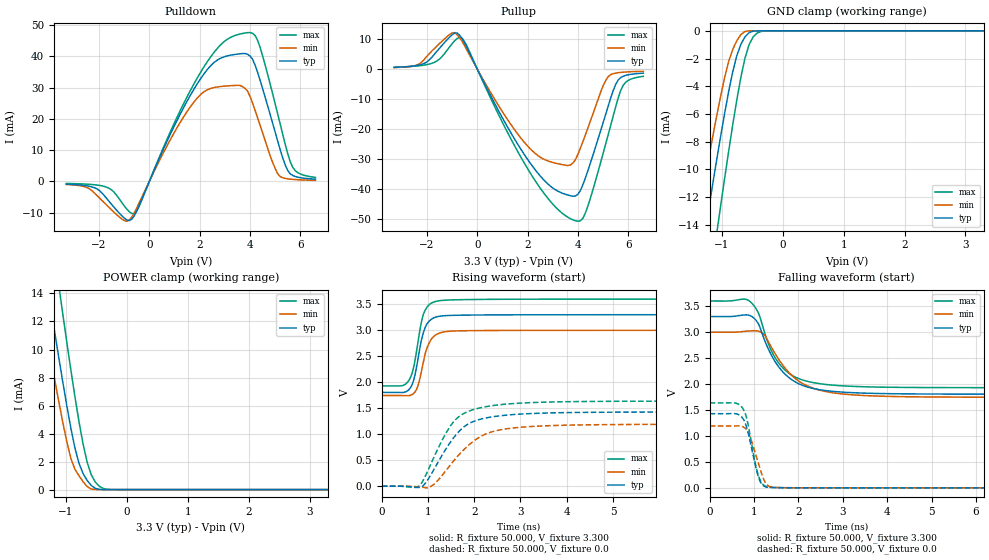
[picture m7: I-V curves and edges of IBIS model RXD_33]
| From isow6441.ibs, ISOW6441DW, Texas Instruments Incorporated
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|   RXD_33 Model
[Model]   RXD_33
Model_type 3-state
| Signals   RXD
Vmeas = 2.2V   |Reference voltage for timing measurements
Cref = 15pF   |Timing specification test load capacitance value
Vref = 0   |Timing specification test load voltage; GND
Polarity   Non-Inverting
Enable   Active-High
C_comp   2.100pF   1.700pF   2.500pF
[Temperature Range]   27.000   -40.000   0.125k
[Voltage Range]   3.300V   3.000V   3.600V
[Pullup Reference]   3.300V   3.000V   3.600V
[Pulldown Reference]   0.0V   0.0V   0.0V
[POWER Clamp Reference]   3.300V   3.000V   3.600V
[GND Clamp Reference]   0.0V   0.0V   0.0V
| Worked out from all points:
|   slope of the pulldown table from 0 to 0.495 V, typ, clamps not added: 54 ohm
|   slope of the pullup table from 0 to 0.495 V, typ, clamps not added: 59.6 ohm
|   GND clamp passes 1 mA (typ) near -0.69 V on its own axis
|   POWER clamp passes 1 mA (typ) near -0.70 V on its own axis
|   rising waveform, R_fixture 50.000, V_fixture 3.300: 20-80 % time 209ps typ, 218ps min, 204ps max; typ from 1.8 V to 3.3 V
|   rising waveform, R_fixture 50.000, V_fixture 0.0: 20-80 % time 673ps typ, 800ps min, 618ps max; typ from 0 V to 1.43 V
|   falling waveform, R_fixture 50.000, V_fixture 3.300: 20-80 % time 647ps typ, 760ps min, 564ps max; typ from 3.3 V to 1.8 V
|   falling waveform, R_fixture 50.000, V_fixture 0.0: 20-80 % time 231ps typ, 262ps min, 225ps max; typ from 1.43 V to 0 V
[Pulldown]
|Voltage   I(typ)   I(min)   I(max)
-3.3V     -873.2uA   -976.9uA   -658.3uA
-1.7V     -5.395mA   -7.539mA   -1.844mA
-900mV    -12.28mA   -12.75mA   -8.801mA
-600mV    -11.02mA   -10.11mA   -10.3mA
2V        32.38mA    27.46mA    34.36mA
3V        39.89mA    30.45mA    44.84mA
4V        40.06mA    27.17mA    47.56mA
4.4V      32.32mA    17.94mA    42.82mA
5.1V      12.87mA    2.427mA    21.53mA
5.5V      3.442mA    821uA      8.827mA
5.8V      1.561mA    581.2uA    3.422mA
6.6V      711uA      333.9uA    1.284mA
[Pullup]
|Voltage   I(typ)   I(min)   I(max)
-3.3V     572.5uA    495.9uA    587.7uA
-2.1V     1.91mA     3.303mA    1.333mA
-1V       11.42mA    12.06mA    8.45mA
-600mV    10.16mA    9.258mA    10.25mA
2.2V      -32.5mA    -27.4mA    -35.95mA
3.6V      -42.06mA   -32.22mA   -49.46mA
4V        -41.78mA   -28.45mA   -50.82mA
4.4V      -33.81mA   -19.56mA   -45.61mA
5.1V      -15.18mA   -3.859mA   -25.08mA
5.5V      -5.127mA   -1.348mA   -12.6mA
5.9V      -2.103mA   -980.9uA   -4.383mA
6.6V      -1.37mA    -744.9uA   -2.434mA
[GND_clamp]
|Voltage   I(typ)   I(min)   I(max)
-3.3V     -72.49mA   -60.83mA   -87.48mA
-1.424V   -18.62mA   -14.18mA   -25.42mA
-1.29V    -14.9mA    -10.95mA   -21.12mA
-1.223V   -13.05mA   -9.358mA   -18.98mA
-1.089V   -9.436mA   -6.249mA   -14.77mA
-1.022V   -7.681mA   -4.767mA   -12.71mA
-821mV    -2.955mA   -1.346mA   -6.782mA
-754mV    -1.794mA   -716.5uA   -4.976mA
-620mV    -433uA     -46.82uA   -1.974mA
-486mV    -22.19uA   -122.9nA   -439.7uA
-352mV    -188.7nA   -149.6pA   -41.75uA
3.3V      0A         0A         0A
[POWER_clamp]
|Voltage   I(typ)   I(min)   I(max)
-3.3V     72.42mA    60.76mA    87.55mA
-1.457V   18.82mA    14.4mA     25.49mA
-1.39V    16.92mA    12.76mA    23.3mA
-1.256V   13.18mA    9.518mA    18.96mA
-1.122V   9.514mA    6.365mA    14.69mA
-1.055V   7.736mA    4.856mA    12.6mA
-921mV    4.407mA    2.239mA    8.56mA
-854mV    2.978mA    1.453mA    6.647mA
-720mV    1.15mA     566.2uA    3.255mA
-586mV    297uA      40.11uA    1.07mA
-318mV    172.9nA    110.5pA    20.56uA
3.3V      0A         0A         0A
[Ramp]
| variable   typ   min   max
dV/dt_r   0.857/0.672n   0.715/0.799n   0.982/0.618n
dV/dt_f   0.897/0.647n   0.753/0.760n   1.002/0.564n
R_load = 50.000
[Rising Waveform]
R_fixture= 50.000
V_fixture= 3.300
V_fixture_min= 3.000
V_fixture_max= 3.600
|time   V(typ)   V(min)   V(max)
0s        1.805V     1.745V     1.93V
432ps     1.803V     1.744V     1.933V
570ps     1.844V     1.742V     2.015V
666ps     1.977V     1.769V     2.205V
767ps     2.362V     1.895V     2.679V
851ps     2.78V      2.179V     3.129V
909ps     2.978V     2.427V     3.328V
1.049ns   3.196V     2.795V     3.509V
1.269ns   3.273V     2.953V     3.572V
15ns      3.3V       3V         3.6V
[Rising Waveform]
R_fixture= 50.000
V_fixture= 0.0
V_fixture_min= 0.0
V_fixture_max= 0.0
|time   V(typ)   V(min)   V(max)
0s        349.6nV    189.3nV    1.057uV
797ps     -25.02mV   -12.81mV   504.4uV
911ps     24.46mV    -24.18mV   138.8mV
1.103ns   283.1mV    19.68mV    508.3mV
1.373ns   696.4mV    283.7mV    995.5mV
1.583ns   964.4mV    516.8mV    1.269V
1.933ns   1.227V     830.1mV    1.46V
2.463ns   1.344V     1.066V     1.558V
4.453ns   1.421V     1.181V     1.63V
15ns      1.428V     1.191V     1.636V
[Falling Waveform]
R_fixture= 50.000
V_fixture= 3.300
V_fixture_min= 3.000
V_fixture_max= 3.600
|time   V(typ)   V(min)   V(max)
0s        3.3V       3V         3.6V
903ps     3.321V     3.023V     3.594V
1.087ns   3.177V     3.021V     3.387V
1.219ns   2.888V     2.96V      3.046V
1.389ns   2.559V     2.712V     2.643V
1.598ns   2.284V     2.422V     2.36V
1.988ns   2.014V     2.067V     2.112V
2.498ns   1.888V     1.878V     2.005V
4.408ns   1.811V     1.756V     1.935V
15ns      1.805V     1.745V     1.93V
[Falling Waveform]
R_fixture= 50.000
V_fixture= 0.0
V_fixture_min= 0.0
V_fixture_max= 0.0
|time   V(typ)   V(min)   V(max)
0s        1.428V     1.191V     1.636V
552ps     1.431V     1.193V     1.637V
739ps     1.348V     1.181V     1.539V
817ps     1.211V     1.134V     1.395V
891ps     975.2mV    1.026V     1.108V
1.027ns   445.4mV    673.4mV    480.8mV
1.1ns     207mV      466.8mV    233.6mV
1.23ns    30.34mV    142mV      45.19mV
1.328ns   10.76mV    37.02mV    14.86mV
15ns      567.6pV    530.8pV    92.41nV
